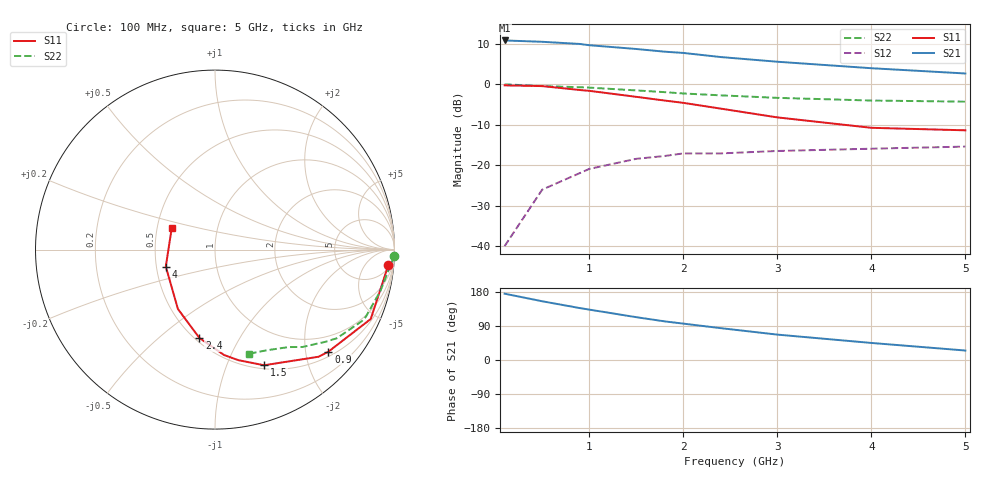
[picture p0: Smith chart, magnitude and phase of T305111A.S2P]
!AT-30511
!S and NOISE PARAMETERS at Vce=1V  Ic=1mA.  LAST UPDATED 06-23-94
# ghz s ma r 50!
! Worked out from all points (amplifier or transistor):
!   11 points, 100 MHz to 5 GHz, reference 50 ohm
!   highest |S21| = 10.8 dB at 100 MHz (marker M1)
!   |S21| within 3 dB of that: start of sweep to 1.947 GHz
!   unconditionally stable (mu >= 1): 3.275 GHz to end of sweep
!   at 500 MHz: K = 0.19, MSG = 18.3 dB, |S12| = -26.0 dB
!   at 1.8 GHz: K = 0.57, MSG = 12.9 dB, |S12| = -17.7 dB
!   at 5 GHz: K = 1.24, MAG = 6.1 dB, |S12| = -15.4 dB
!   lowest NFmin = 0.30 dB at 500 MHz
!   S11 on the Smith chart (normalised r, x): 100 MHz: 7, -20; 900 MHz: 0.60, -2.48; 1.5 GHz: 0.54, -1.37; 2.4 GHz: 0.53, -0.69; 4 GHz: 0.56, -0.12; 5 GHz: 0.60, +0.16
0.1  0.97 -5.0  3.48 175.0  0.01 86.0  0.999 -2.0
0.5  0.95 -24.0  3.35 155.0  0.05 72.0  0.95 -14.0
0.9  0.85 -42.0  3.15 137.0  0.08 61.0  0.92 -24.0
1  0.83 -46.0  3.04 133.0  0.09 58.0  0.91 -26.0
1.5  0.7 -67.0  2.73 113.0  0.12 46.0  0.84 -36.0
1.8  0.63 -78.0  2.53 102.0  0.13 41.0  0.8 -40.0
2  0.59 -85.0  2.44 96.0  0.14 37.0  0.77 -43.0
2.4  0.5 -100.0  2.17 84.0  0.14 32.0  0.73 -48.0
3  0.39 -122.0  1.9 67.0  0.15 27.0  0.68 -53.0
4  0.29 -161.0  1.58 45.0  0.16 20.0  0.63 -63.0
5  0.27 153.0  1.36 25.0  0.17 20.0  0.61 -72.0
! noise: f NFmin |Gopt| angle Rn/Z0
0.5  0.3  0.96  10  1.49
0.9  0.4  0.92  19  1.33
1.8  0.9  0.83  43  0.98
2.4  1.3  0.76  60  0.74
